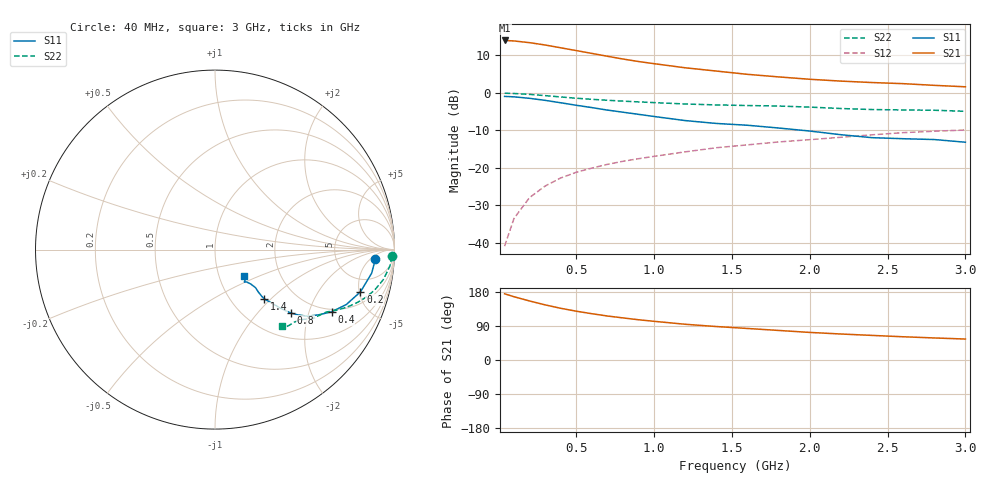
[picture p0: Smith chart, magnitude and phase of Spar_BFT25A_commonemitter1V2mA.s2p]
! Filename:  BFT25AE.S2P  Version:  2.0
! NXP part #: BFT25A  Date: Aug 1990
! Bias condition: Vce=1V, Ic=2mA
#  MHz  S  MA  R  50
! Freq  S11  S21  S12  S22  !GUM [dB]
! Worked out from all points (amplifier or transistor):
!   21 points, 40 MHz to 3 GHz, reference 50 ohm
!   highest |S21| = 14.0 dB at 40 MHz (marker M1)
!   |S21| within 3 dB of that: start of sweep to 540.1 MHz
!   unconditionally stable (mu >= 1): 1.547 GHz to end of sweep
!   at 300 MHz: K = 0.39, MSG = 18.8 dB, |S12| = -24.9 dB
!   at 1 GHz: K = 0.86, MSG = 12.4 dB, |S12| = -17.0 dB
!   at 3 GHz: K = 1.15, MAG = 3.4 dB, |S12| = -9.9 dB
!   S11 on the Smith chart (normalised r, x): 40 MHz: 14, -7; 200 MHz: 3.15, -5.15; 400 MHz: 1.88, -2.85; 800 MHz: 1.52, -1.54; 1.4 GHz: 1.41, -0.92; 3 GHz: 1.32, -0.41
40  0.895 -3.4  4.989 174.7  0.009 85.4  0.987 -2.2
100  0.883 -8.5  4.915 167.0  0.021 84.9  0.979 -5.4
200  0.844 -16.2  4.662 155.8  0.04 80.0  0.952 -10.2
300  0.793 -22.7  4.342 145.5  0.057 76.1  0.917 -14.3
400  0.736 -28.1  3.984 136.5  0.073 73.2  0.88 -17.7
500  0.682 -32.2  3.657 128.8  0.087 71.6  0.847 -20.3
600  0.635 -35.8  3.353 122.2  0.099 70.2  0.818 -22.4
700  0.588 -38.2  3.07 116.1  0.111 69.1  0.795 -24.0
800  0.551 -39.9  2.821 111.1  0.122 68.3  0.774 -25.3
900  0.516 -41.0  2.613 106.2  0.132 67.6  0.756 -26.5
1000  0.483 -42.0  2.445 102.1  0.142 66.9  0.74 -27.4
1200  0.426 -43.6  2.155 94.3  0.163 65.6  0.709 -29.5
1400  0.39 -45.0  1.949 88.3  0.185 64.7  0.689 -32.0
1600  0.369 -45.0  1.763 83.2  0.202 63.9  0.676 -33.7
1800  0.339 -44.4  1.629 78.0  0.221 63.0  0.666 -35.4
2000  0.309 -43.2  1.515 72.8  0.237 61.5  0.644 -36.9
2200  0.276 -43.9  1.432 68.6  0.255 60.1  0.617 -39.3
2400  0.252 -45.7  1.37 64.9  0.275 58.6  0.598 -42.6
2600  0.244 -47.9  1.324 61.3  0.294 57.3  0.59 -45.8
2800  0.238 -45.4  1.257 58.2  0.307 56.7  0.585 -47.4
3000  0.219 -41.9  1.202 55.3  0.319 56.1  0.566 -48.4
